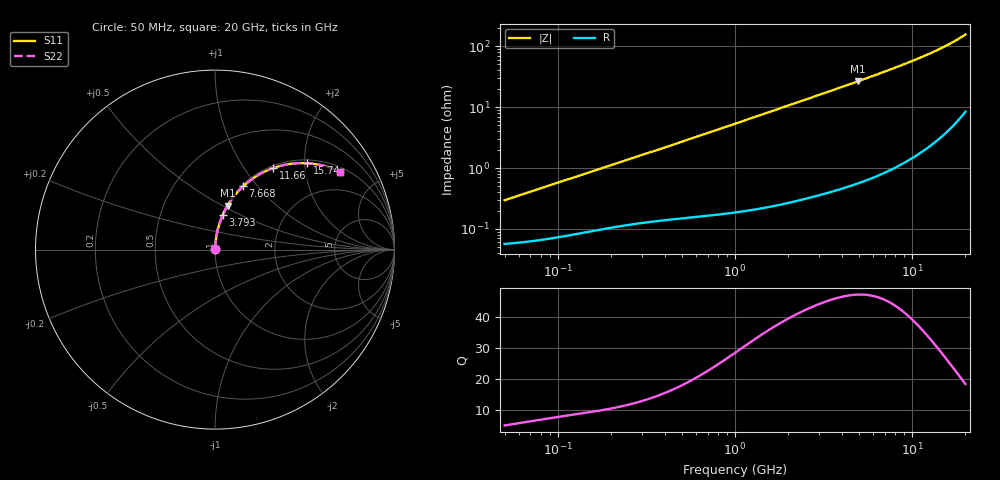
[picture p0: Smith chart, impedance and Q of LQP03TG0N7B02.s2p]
!Murata Part Number: LQP03TG0N7B02
!These Parameters are Measured in Series Mode Connection
!  o--[Z]--o
!Port1  Port2
!  o-------o
!Freq. Start=50[MHz] Stop=20[GHz], 401[Steps]
# Hz S RI R 50
!Freq.(Hz) S11(Real) S11(Imag) S21(Real) S21(Imag) S12(Real) S12(Imag) S22(Real) S22(Imag)
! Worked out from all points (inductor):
!   401 points, 50 MHz to 20 GHz, reference 50 ohm
!   read as one part in series: L = 922 pH near 51.52 MHz
!   highest Q = 47.4 at 4.967 GHz (marker M1), where L = 851 pH
!   S11 on the Smith chart (normalised r, x): 50 MHz: 1.00, +0.01; 3.793 GHz: 1.01, +0.40; 7.668 GHz: 1.02, +0.84; 11.66 GHz: 1.04, +1.37; 15.74 GHz: 1.08, +2.06; 20 GHz: 1.17, +3.10
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5e7  0.000576 0.0029  0.9994 -0.0029  0.9994 -0.0029  0.000576 0.0029
5.152053e7  0.00058 0.00299  0.9994 -0.00299  0.9994 -0.00299  0.00058 0.00299
1.364002e8  0.000915 0.0077  0.9991 -0.0077  0.9991 -0.0077  0.000915 0.0077
3.721004e8  0.00176 0.0201  0.9982 -0.0201  0.9982 -0.0201  0.00176 0.0201
6.380365e8  0.00276 0.034  0.9972 -0.034  0.9972 -0.034  0.00276 0.034
1e9  0.00466 0.0528  0.9953 -0.0528  0.9953 -0.0528  0.00466 0.0528
1.714689e9  0.0106 0.0897  0.9894 -0.0897  0.9894 -0.0897  0.0106 0.0897
2.728004e9  0.0236 0.1407  0.9764 -0.1407  0.9764 -0.1407  0.0236 0.1407
3.792786e9  0.0429 0.1921  0.9571 -0.1921  0.9571 -0.1921  0.0429 0.1921
4.966507e9  0.0705 0.2456  0.9295 -0.2456  0.9295 -0.2456  0.0705 0.2456
6.125241e9  0.1038 0.2945  0.8962 -0.2945  0.8962 -0.2945  0.1038 0.2945
7.442007e9  0.1481 0.3443  0.8519 -0.3443  0.8519 -0.3443  0.1481 0.3443
7.668323e9  0.1564 0.3522  0.8436 -0.3522  0.8436 -0.3522  0.1564 0.3522
8.516016e9  0.1888 0.3798  0.8112 -0.3798  0.8112 -0.3798  0.1888 0.3798
9.457416e9  0.2272 0.4069  0.7728 -0.4069  0.7728 -0.4069  0.2272 0.4069
1.050288e10  0.2723 0.4322  0.7277 -0.4322  0.7277 -0.4322  0.2723 0.4322
1.166392e10  0.3247 0.4543  0.6753 -0.4543  0.6753 -0.4543  0.3247 0.4543
1.375312e10  0.4222 0.4778  0.5778 -0.4778  0.5778 -0.4778  0.4222 0.4778
1.573793e10  0.5149 0.4812  0.4851 -0.4812  0.4851 -0.4812  0.5149 0.4812
1.774144e10  0.6046 0.4672  0.3954 -0.4672  0.3954 -0.4672  0.6046 0.4672
1.940974e10  0.6741 0.4438  0.3259 -0.4438  0.3259 -0.4438  0.6741 0.4438
2e10  0.6972 0.4333  0.3028 -0.4333  0.3028 -0.4333  0.6972 0.4333
